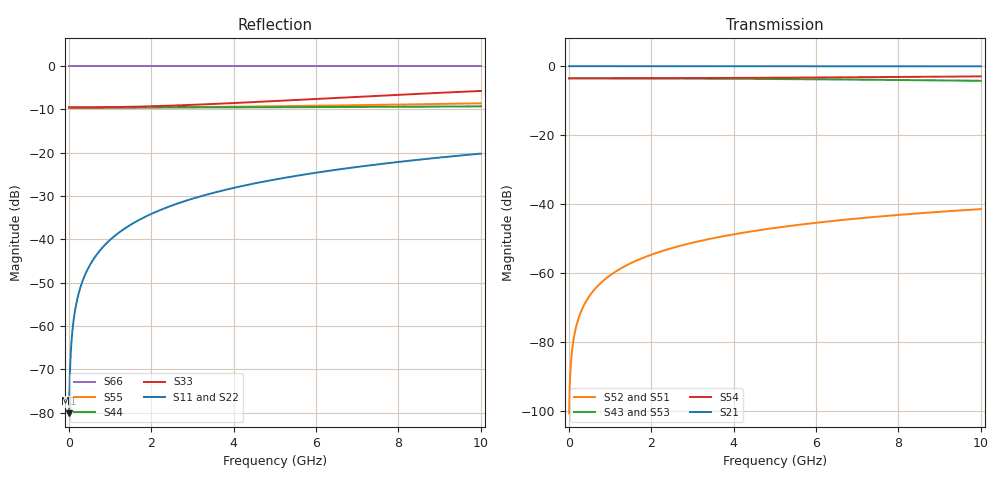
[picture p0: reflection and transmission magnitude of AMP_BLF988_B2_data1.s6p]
! Created Tue Nov 05 10:27:32 2013
# ghz S ma R 50
! 6 Port Network Data from SP1.SP block
! freq  magS11  angS11  magS12  angS12  magS13  angS13  magS14  angS14
!  magS15  angS15  magS16  angS16
!  magS21  angS21  magS22  angS22
!  magS23  angS23  magS24  angS24  magS25  angS25  magS26  angS26
!  magS31  angS31  magS32  angS32  magS33  angS33  magS34  angS34
!  magS35  angS35  magS36  angS36
!  magS41  angS41  magS42  angS42
!  magS43  angS43  magS44  angS44  magS45  angS45  magS46  angS46
!  magS51  angS51  magS52  angS52  magS53  angS53  magS54  angS54
!  magS55  angS55  magS56  angS56
!  magS61  angS61  magS62  angS62
!  magS63  angS63  magS64  angS64  magS65  angS65  magS66  angS66
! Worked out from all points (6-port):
!   1000 points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, 10 MHz to 10 GHz, reference 50 ohm
!   strongest paths, dB at 10 MHz, 2.51 GHz, 5.01 GHz, 7.51 GHz, 10 GHz:
!     S21: 0.0, 0.0, 0.0, 0.0, 0.0
!     S54: -3.5, -3.5, -3.3, -3.2, -3.0
!     S43: -3.5, -3.6, -3.7, -4.0, -4.2
!     S53: -3.5, -3.6, -3.8, -4.1, -4.5
!     S52: -100.7, -52.7, -46.9, -43.6, -41.5
!     S51: -100.7, -52.7, -46.9, -43.6, -41.5
!   lowest |S11| = -80.1 dB at 10 MHz (marker M1), VSWR 1.00, Z = 50 + j0.00984 ohm
!   |S11| at or under -10 dB: start of sweep to end of sweep
